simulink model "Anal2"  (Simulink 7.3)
settings: Solver=ode45  StartTime=0.0  StopTime=10.0  RelTol=1e-3
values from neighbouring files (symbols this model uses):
  Kl3 = INFO.KFI(:,1:7)    [run.m]
  Kp = om^2    (= 1)    [run.m]
  Kr = 2*zt*om    (= 0.28)    [run.m]
undefined symbols (not defined in the file or in its folder): An, Bn, Cn, Dn

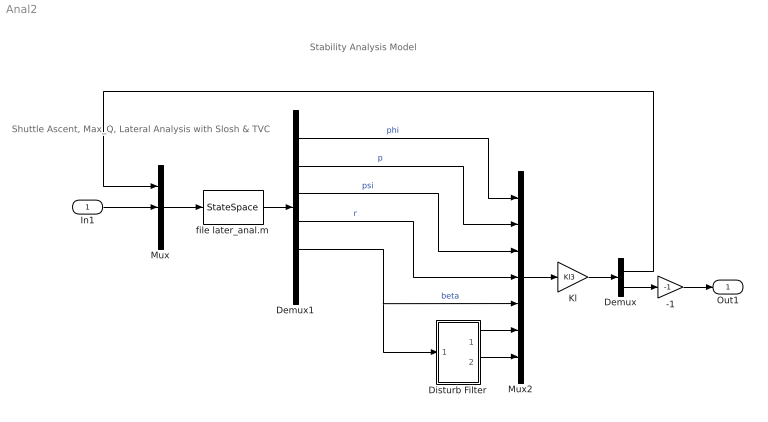
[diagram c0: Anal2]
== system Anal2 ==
  note: Shuttle Ascent, Max_Q, Lateral Analysis with Slosh & TVC
  note: Stability Analysis Model
  In1 : Inport  OutDataType=sfix(16)  OutScaling=2^0
  -1 : Gain  Gain=-1  ParameterDataType=sfix(16)  ParameterScaling=2^0  OutDataType=sfix(16)  OutScaling=2^0
  Demux : Demux  Outputs=2
  Demux1 : Demux  Outputs=6
  Disturb Filter : Subsystem
  Kl : Gain  Gain=Kl3  Multiplication=Matrix(K*u)  ParameterDataType=sfix(16)  ParameterScaling=2^0  OutDataType=sfix(16)  OutScaling=2^0
  Mux : Mux  Inputs=3
  Mux2 : Mux  Inputs=7
  file later_anal.m : StateSpace  A=An  B=Bn  C=Cn  D=Dn
  Out1 : Outport  OutDataType=sfix(16)  OutScaling=2^0
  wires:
  Mux/1 -> file later_anal.m/1
  Kl/1 -> Demux/1
  -1/1 -> Out1/1
  In1/1 -> Mux/2
  Demux/2 -> -1/1
  Demux/1 -> Mux/1
  file later_anal.m/1 -> Demux1/1
  Mux2/1 -> Kl/1
  Disturb Filter/1(x1) -> Mux2/6
  Disturb Filter/2(x2) -> Mux2/7
  Demux1/1 -> Mux2/1  "phi"
  Demux1/2 -> Mux2/2  "p"
  Demux1/3 -> Mux2/3  "psi"
  Demux1/4 -> Mux2/4  "r"
  Demux1/5 -> Mux2/5, Disturb Filter/1(bet)  "beta"

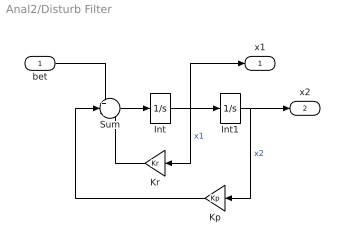
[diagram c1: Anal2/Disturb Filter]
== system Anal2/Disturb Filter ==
  bet : Inport  OutDataType=sfix(16)  OutScaling=2^0
  Int : Integrator
  Int1 : Integrator
  Kp : Gain  Gain=Kp  ParameterDataType=sfix(16)  ParameterScaling=2^0  OutDataType=sfix(16)  OutScaling=2^0
  Kr : Gain  Gain=Kr  ParameterDataType=sfix(16)  ParameterScaling=2^0  OutDataType=sfix(16)  OutScaling=2^0
  Sum : Sum  Inputs=+--  OutDataType=sfix(16)  OutScaling=2^0
  x1 : Outport  OutDataType=sfix(16)  OutScaling=2^0
  x2 : Outport  Port=2  OutDataType=sfix(16)  OutScaling=2^0
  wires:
  Int/1 -> Int1/1, Kr/1, x1/1  "x1"
  Sum/1 -> Int/1
  Int1/1 -> Kp/1, x2/1  "x2"
  Kr/1 -> Sum/3
  Kp/1 -> Sum/2
  bet/1 -> Sum/1
